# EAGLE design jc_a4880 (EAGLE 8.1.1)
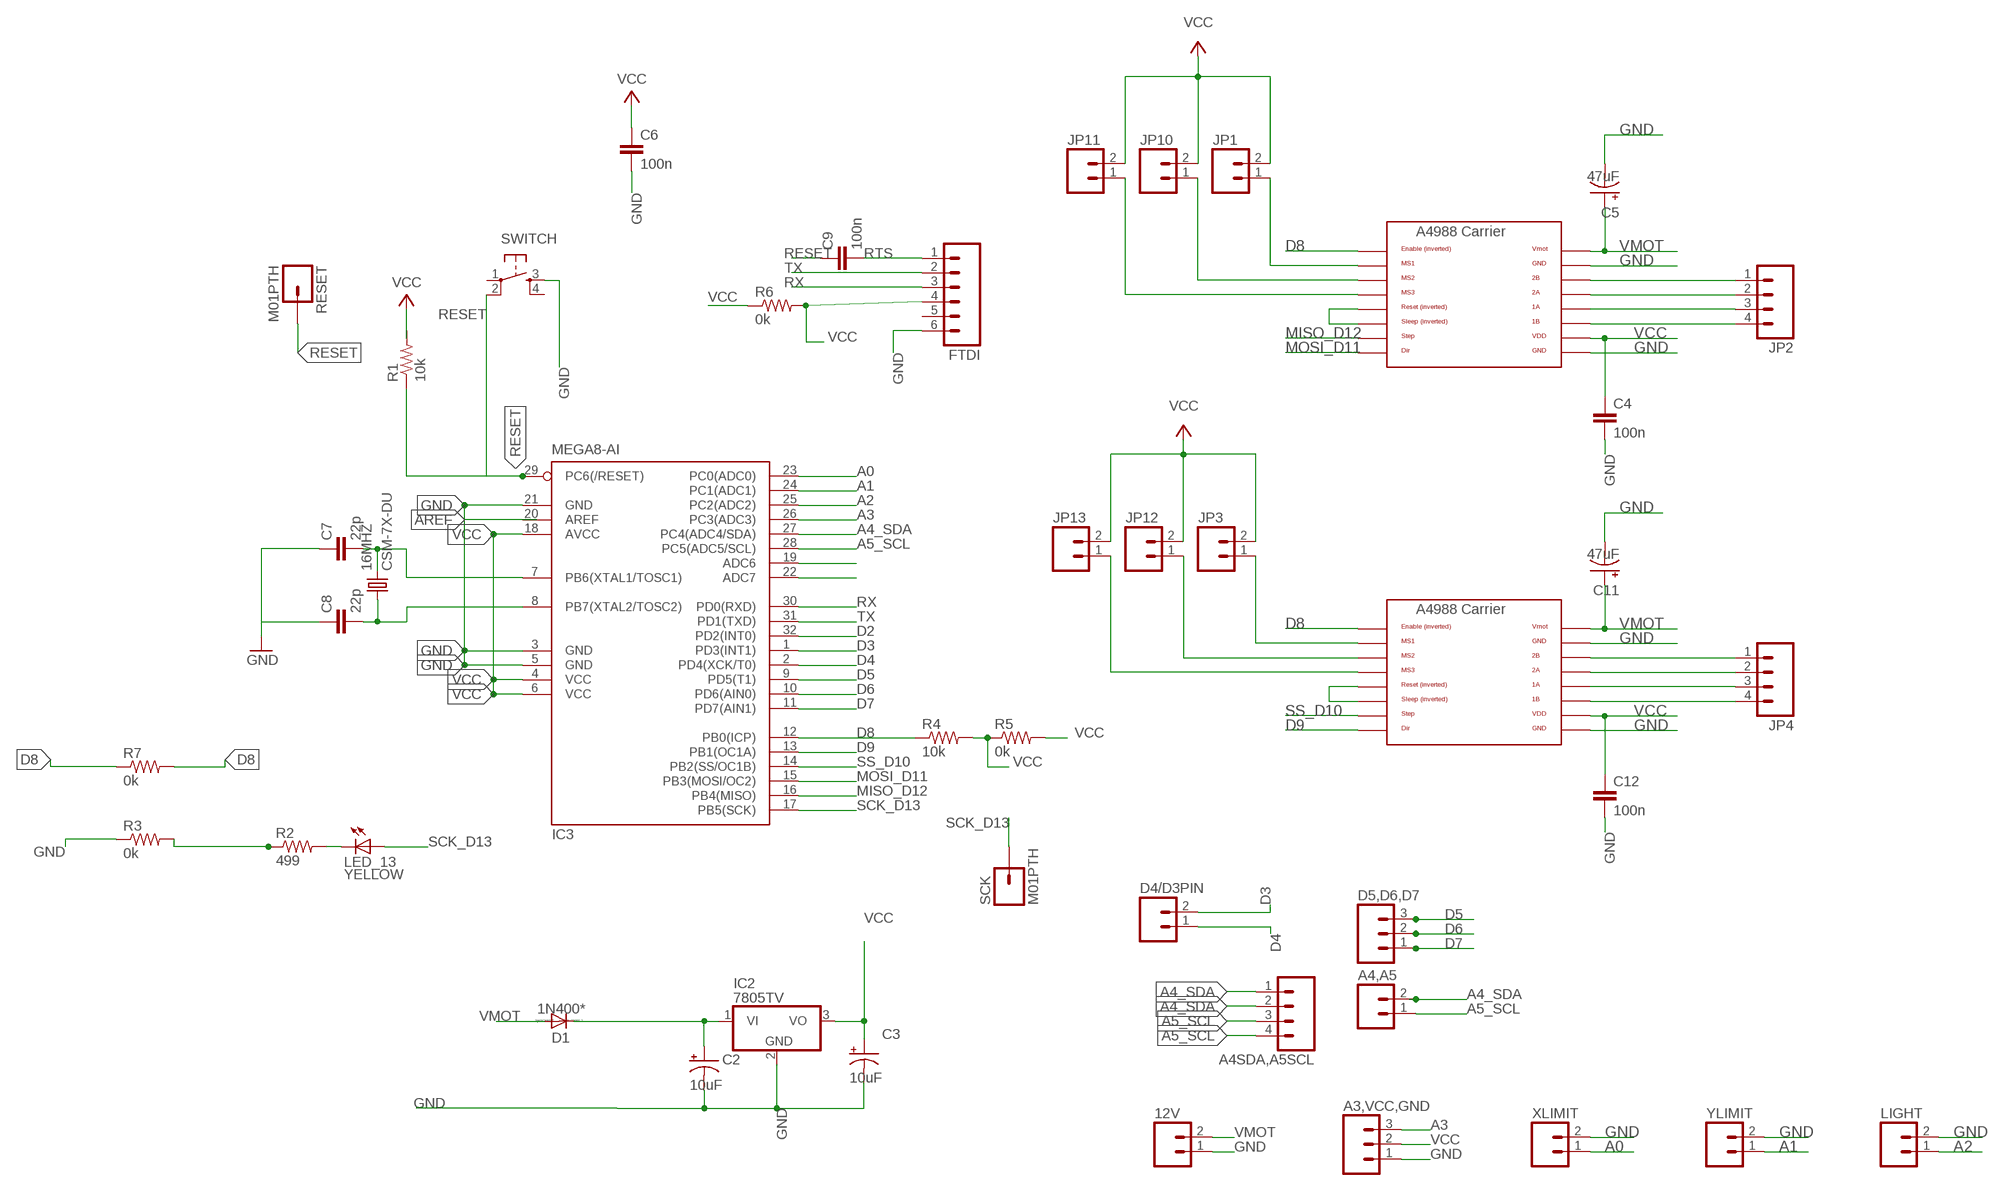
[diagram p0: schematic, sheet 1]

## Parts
12V  M023.5MM_LOCK  [SCREWTERMINAL-3.5MM-2_LOCK]
16MHZ  CSM-7X-DU  [CSM-7X-DU]
A3,VCC,GND  M03PTH  [1X03]
A4,A5  M02PTH  [1X02]
A4SDA,A5SCL  M04PTH  [1X04]
C2  10uF  MCGPR50V107M8X11  [MCGPR50V107M8X11]
C3  10uF  MCGPR50V107M8X11  [MCGPR50V107M8X11]
C4  100n  CAP1206  [1206]
C5  47uF  MCGPR50V107M8X11  [MCGPR50V107M8X11]
C6  100n  CAP1206  [1206]
C7  22p  CAP1206  [1206]
C8  22p  CAP1206  [1206]
C9  100n  CAP1206  [1206]
C11  47uF  MCGPR50V107M8X11  [MCGPR50V107M8X11]
C12  100n  CAP1206  [1206]
D1  1N400*  1N4148DO35-10  [DO35-10]
D4/D3PIN  M02PTH  [1X02]
D5,D6,D7  M03PTH  [1X03]
FTDI  M06LONGPADS  [1X06_LONGPADS]
IC2  7805TV  [TO220V]
IC3  MEGA8-AI  [TQFP32-08]
JP1  M02PTH  [1X02]
JP2  M04PTH  [1X04]
JP3  M02PTH  [1X02]
JP4  M04PTH  [1X04]
JP10  M02PTH  [1X02]
JP11  M02PTH  [1X02]
JP12  M02PTH  [1X02]
JP13  M02PTH  [1X02]
LED_13  YELLOW  LED1206  [1206]
LIGHT  M02LOCK_LONGPADS  [1X02_LOCK_LONGPADS]
R1  10k  RESISTOR1206  [1206]
R2  499  RESISTOR1206  [1206]
R3  0k  RESISTOR1206  [1206]
R4  10k  RESISTOR1206  [1206]
R5  0k  RESISTOR1206  [1206]
R6  0k  RESISTOR1206  [1206]
R7  0k  RESISTOR1206  [1206]
RESET  M01PTH  [1X01]
SCK  M01PTH  [1X01]
SWITCH  6MM_SWITCH6MM_SWITCH  [6MM_SWITCH]
XAXIS  A4988BREAKOUT  [A4988BREAKOUT]
XLIMIT  M02LOCK_LONGPADS  [1X02_LOCK_LONGPADS]
YAXIS1  A4988BREAKOUT  [A4988BREAKOUT]
YLIMIT  M02LOCK_LONGPADS  [1X02_LOCK_LONGPADS]

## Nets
A0: IC3.23(PC0(ADC0)) XLIMIT.1
A1: IC3.24(PC1(ADC1)) YLIMIT.1
A2: IC3.25(PC2(ADC2)) LIGHT.1
A3: A3,VCC,GND.3 IC3.26(PC3(ADC3))
A4_SDA: A4,A5.2 A4SDA,A5SCL.1 A4SDA,A5SCL.2 IC3.27(PC4(ADC4/SDA))
A5_SCL: A4,A5.1 A4SDA,A5SCL.3 A4SDA,A5SCL.4 IC3.28(PC5(ADC5/SCL))
AREF [aref]: IC3.20(AREF)
D2: IC3.32(PD2(INT0))
D3: D4/D3PIN.2 IC3.1(PD3(INT1))
D4: D4/D3PIN.1 IC3.2(PD4(XCK/T0))
D5: D5,D6,D7.3 IC3.9(PD5(T1))
D6: D5,D6,D7.2 IC3.10(PD6(AIN0))
D7: D5,D6,D7.1 IC3.11(PD7(AIN1))
D8: IC3.12(PB0(ICP)) R4.1 R7.1 R7.2 XAXIS.EN YAXIS1.EN
D9: IC3.13(PB1(OC1A)) YAXIS1.DIR
GND: 12V.1 A3,VCC,GND.1 C2.- C3.- C4.2 C5.- C6.2 C7.1 C8.1 C11.- C12.2 FTDI.6 IC2.2(GND) IC3.3(GND) IC3.5(GND) IC3.21(GND) LIGHT.2 R2.1 R3.1 R3.2 SWITCH.3(S) XAXIS.GND XAXIS.GND@0(GND) XLIMIT.2 YAXIS1.GND YAXIS1.GND@0(GND) YLIMIT.2
MISO_D12: IC3.16(PB4(MISO)) XAXIS.STEP
MOSI_D11: IC3.15(PB3(MOSI/OC2)) XAXIS.DIR
N$2: XAXIS.RST XAXIS.SLP(SLEEP)
N$3: JP1.1 XAXIS.MS1
N$4: JP10.1 XAXIS.MS2
N$5: JP11.1 XAXIS.MS3
N$6: 16MHZ.1 C8.2 IC3.8(PB7(XTAL2/TOSC2))
N$8: 16MHZ.2 C7.2 IC3.7(PB6(XTAL1/TOSC1))
N$9: JP2.1 XAXIS.2B
N$10: JP2.2 XAXIS.2A
N$11: JP2.3 XAXIS.1A
N$12: JP2.4 XAXIS.1B
N$13: YAXIS1.RST YAXIS1.SLP(SLEEP)
N$16: JP13.1 YAXIS1.MS3
N$18: JP4.2 YAXIS1.2A
N$19: JP4.1 YAXIS1.2B
N$20: JP4.3 YAXIS1.1A
N$21: JP4.4 YAXIS1.1B
N$27: LED_13.2(C) R2.2
N$38: IC3.22(ADC7)
N$39: IC3.19(ADC6)
N$54: JP3.1 YAXIS1.MS1
N$55: JP12.1 YAXIS1.MS2
RESET: C9.1 IC3.29(PC6(/RESET)) R1.1 RESET.1 SWITCH.2(P1)
RTS: C9.2 FTDI.1
RX: FTDI.3 IC3.30(PD0(RXD))
SCK_D13: IC3.17(PB5(SCK)) LED_13.1(A) SCK.1
SS_D10: IC3.14(PB2(SS/OC1B)) YAXIS1.STEP
TX: FTDI.2 IC3.31(PD1(TXD))
V_IN [gnd]: C2.+ D1.C IC2.1(VI)
VCC: A3,VCC,GND.2 C3.+ C4.1 C6.1 C12.1 FTDI.4 IC2.3(VO) IC3.4(VCC) IC3.6(VCC) IC3.18(AVCC) JP1.2 JP3.2 JP10.2 JP11.2 JP12.2 JP13.2 R1.2 R4.2 R5.1 R5.2 R6.1 R6.2 XAXIS.VDD YAXIS1.VDD
VMOT: 12V.2 C5.+ C11.+ D1.A XAXIS.VMOT YAXIS1.VMOT
Unconnected: FTDI.5 SWITCH.1(P) SWITCH.4(S1)

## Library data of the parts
12V = 01_SparkFun:M02: Header 2
16MHZ = 01_FAB_Hello:CSM-7X-DU: SMD CRYSTAL; OC_FARNELL: unknown; OC_NEWARK: unknown
A3,VCC,GND D5,D6,D7 = 01_SparkFun:M03: Header 3 Standard 3-pin 0.1" header. Use with straight break away headers (SKU : PRT-00116), right angle break away headers (PRT-00553), swiss pins (PRT-00743), machine pins (PRT-00117), and female headers (PRT-00115). Molex polarized connector foot print use with SKU : PRT-08232 with associated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
A4,A5 D4/D3PIN JP1 JP3 JP10-JP13 LIGHT XLIMIT YLIMIT = SparkFun-Connectors:M02: Header 2
A4SDA,A5SCL JP2 JP4 = SparkFun-Connectors:M04: Header 4 Standard 4-pin 0.1" header. Use with straight break away headers (SKU : PRT-00116), right angle break away headers (PRT-00553), swiss pins (PRT-00743), machine pins (PRT-00117), and female headers (PRT-00115). Molex polarized connector foot print use with SKU : PRT-08231 with associated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
C2 C3 C5 C11 = Ryan:MCGPR50V107M8X11
C4 C6-C9 C12 = 01_SparkFun:CAP: Capacitor
D1 = diode:1N4148: DIODE
FTDI = 01_SparkFun:M06: Header 6 Standard 6-pin 0.1" header. Use with straight break away headers (SKU : PRT-00116), right angle break away headers (PRT-00553), swiss pins (PRT-00743), machine pins (PRT-00117), and female headers (PRT-00115). Molex polarized connector foot print use with SKU : PRT-08094 with associated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
IC2 = linear:78*: Positive VOLTAGE REGULATOR Source: http://cache.national.com/ds/LM/LM78L05.pdf http://www.fairchildsemi.com/ds/LM/LM7805.pdf
IC3 = 01_atmel:MEGA8: MICROCONTROLLER 8 Kbytes FLASH, 1 kbytes SRAM, 512 bytes EEPROM, USART, 6-channel 10 bit ADC, 2-channel 8 bit ADC Pin compatible with Atmega48, ATMega88, ATMega168 Source: avr.lbr
LED_13 = 01_FAB_Hello:LED
R1-R7 = 01_SparkFun:RESISTOR: Resistor
RESET SCK = 01_SparkFun:M01: Header 1
SWITCH = 01_FAB_Hello:6MM_SWITCH: OMRON SWITCH
XAXIS YAXIS1 = RepRapjr:A4988BREAKOUT

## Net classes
0 default: width 0.254 mm, drill 0.254 mm, clearance 0.254 mm
1 power: width 0.254 mm, drill 0.254 mm, clearance 0.254 mm
2 gnd: width 0.254 mm, drill 0.254 mm, clearance 0.254 mm
3 usbvcc: width 0.254 mm, drill 0.254 mm, clearance 0.254 mm
4 aref: width 0.254 mm, drill 0.254 mm, clearance 0.254 mm

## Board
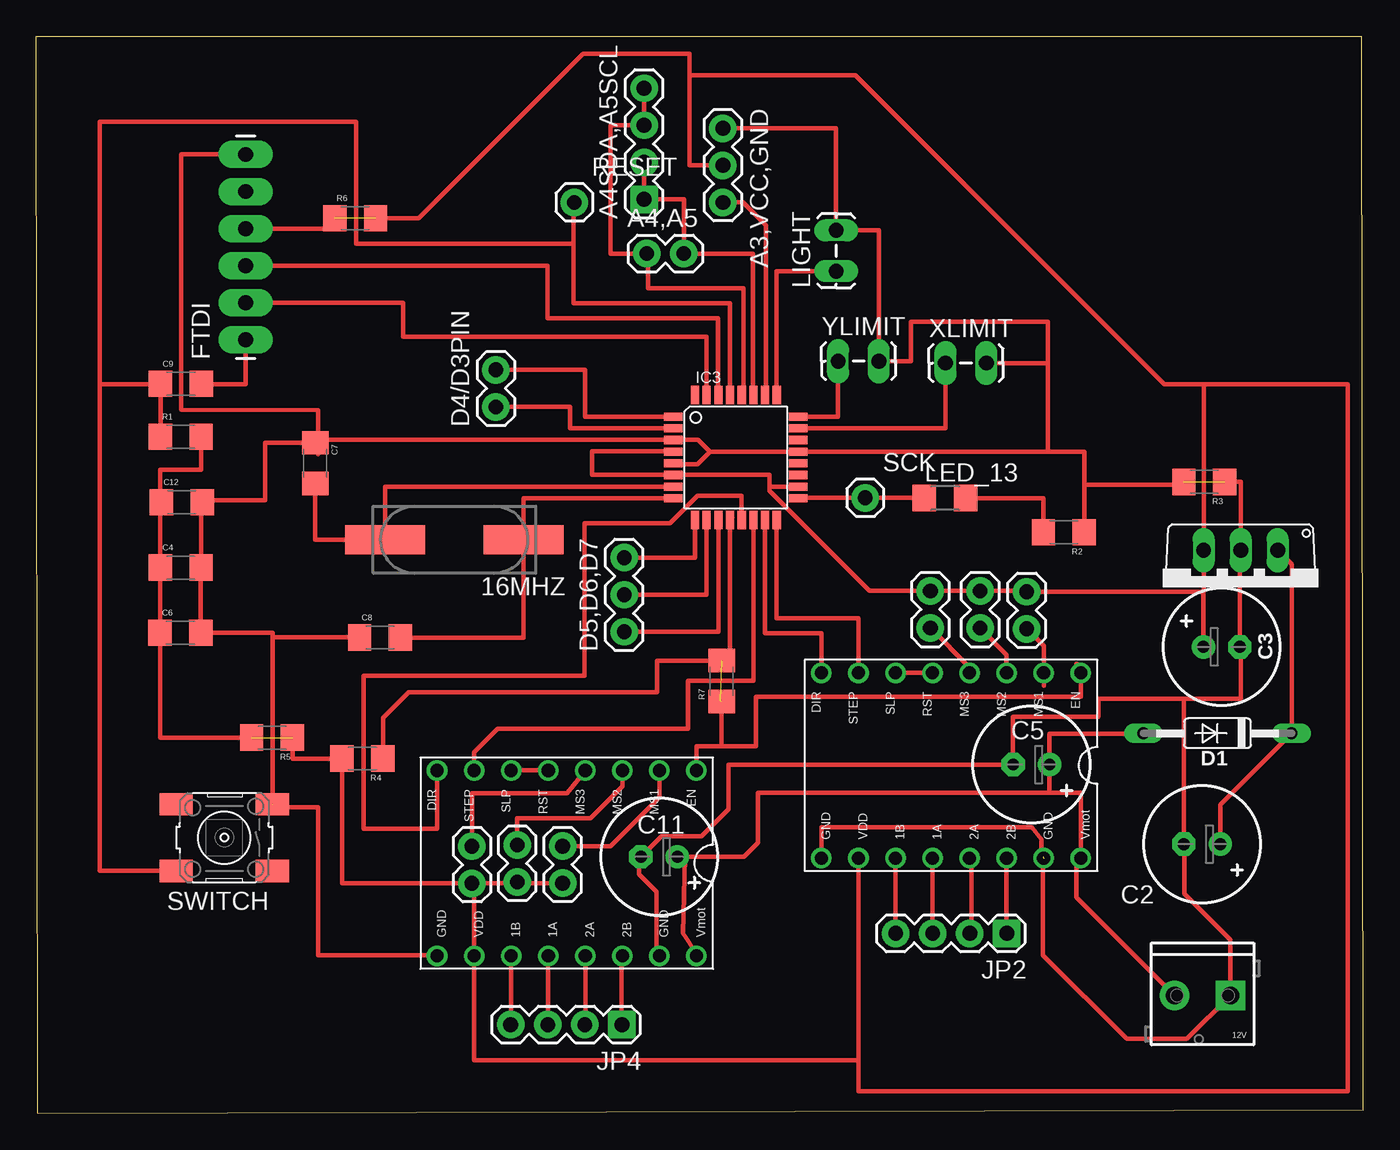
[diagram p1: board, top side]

Size 90.94 x 73.8 mm. Coordinates in mm from the lower left corner, seen from the top.
Outline: 0.09,0 90.94,0.25 90.86,73.8 0,73.8 0.09,0
Copper layers (1*16): Top 0.035mm / dielectric 1.5mm / Bottom 0.035mm
Design rules "default": minimum track width 10mil, minimum drill 24mil, track to track 10mil, track to pad 10mil, pad to pad 10mil, via to via 10mil, smd to smd 10mil, copper to edge 40mil, drill to drill 10mil, minimum pad ring 10mil, minimum via ring 8mil, stop-mask expansion 0mil, vias tented up to drill 0mil, thermal gap 10mil

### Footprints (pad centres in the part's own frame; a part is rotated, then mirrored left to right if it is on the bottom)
SCREWTERMINAL-3.5MM-2_LOCK = drill 1.2 pad 2.032 square: 1 -0.178,0 | drill 1.2 pad 2.032: 2 3.678,0
CSM-7X-DU = smd 5.5 x 2: 1 -4.75,0; 2 4.75,0
1X03 = drill 1.016 pad 1.88: 1 0,0; 2 2.54,0; 3 5.08,0
1X02 = drill 1.016 pad 1.88: 1 0,0; 2 2.54,0
1X04 = drill 1.016 pad 1.88 square: 1 0,0 | drill 1.016 pad 1.88: 2 2.54,0; 3 5.08,0; 4 7.62,0
MCGPR50V107M8X11 = drill 0.813 pad 1.6: + -1.25,0 | drill 0.813 pad 1.6 octagon: - 1.25,0
1206 = smd 1.6 x 1.8: 1 -1.4,0; 2 1.4,0
DO35-10 = drill 0.813 long: A 5.08,0; C -5.08,0
1X06_LONGPADS = drill 1.016 pad 1.88 long: 1 0,0; 2 2.54,0; 3 5.08,0; 4 7.62,0; 5 10.16,0; 6 12.7,0
TO220V = drill 1.016 long: 1 -2.54,-2.54; 2 0,-2.54; 3 2.54,-2.54
TQFP32-08 = smd 1.27 x 0.559: 1 -4.293,2.8; 2 -4.293,2; 3 -4.293,1.2; 4 -4.293,0.4; 5 -4.293,-0.4; 6 -4.293,-1.2; 7 -4.293,-2; 8 -4.293,-2.8; 17 4.293,-2.8; 18 4.293,-2; 19 4.293,-1.2; 20 4.293,-0.4; 21 4.293,0.4; 22 4.293,1.2; 23 4.293,2; 24 4.293,2.8 | smd 0.559 x 1.27: 9 -2.8,-4.293; 10 -2,-4.293; 11 -1.2,-4.293; 12 -0.4,-4.293; 13 0.4,-4.293; 14 1.2,-4.293; 15 2,-4.293; 16 2.8,-4.293; 25 2.8,4.293; 26 2,4.293; 27 1.2,4.293; 28 0.4,4.293; 29 -0.4,4.293; 30 -1.2,4.293; 31 -2,4.293; 32 -2.8,4.293
1206' = smd 1.6 x 1.803: 1 -1.422,0; 2 1.422,0
1X02_LOCK_LONGPADS = drill 1.016 long: 1 -0.127,0; 2 2.667,0
1X01 = drill 1.016 pad 1.88: 1 0,0
6MM_SWITCH = smd 2.286 x 1.524: 1 -3.302,2.286; 2 3.302,2.286; 3 -3.302,-2.286; 4 3.302,-2.286
A4988BREAKOUT = drill 0.9: 1A 8.89,1.27; 1B 11.43,1.27; 2A 6.35,1.27; 2B 3.81,1.27; DIR 16.51,-11.43; EN -1.27,-11.43; GND 16.51,1.27; GND@0 1.27,1.27; MS1 1.27,-11.43; MS2 3.81,-11.43; MS3 6.35,-11.43; RST 8.89,-11.43; SLP 11.43,-11.43; STEP 13.97,-11.43; VDD 13.97,1.27; VMOT -1.27,1.27

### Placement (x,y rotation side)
12V  81.69,8.09 180 top
16MHZ  28.65,39.31 180 top
A3,VCC,GND  47.06,67.5 270 top
A4,A5  41.84,58.92 0 top
A4SDA,A5SCL  41.66,62.63 90 top
C2  79.91,18.45 180 top
C3  81.25,31.97 0 top
C4  9.89,37.41 0 top
C5  68.21,23.9 180 top
C6  9.87,32.94 0 top
C7  19.12,44.56 270 top
C8  23.55,32.61 0 top
C9  9.91,49.99 0 top
C11  42.69,17.58 180 top
C12  9.97,41.89 0 top
D1  80.97,26.04 180 top
D4/D3PIN  31.5,48.41 90 top
D5,D6,D7  40.29,33 90 top
FTDI  14.34,53.01 90 top
IC2  82.55,36.05 180 top
IC3  47.95,44.95 0 top
JP1  67.88,33.2 90 top
JP2  66.52,12.34 180 top
JP3  36.07,18.32 270 top
JP4  40.13,6.08 180 top
JP10  64.7,33.26 90 top
JP11  61.28,33.26 90 top
JP12  32.96,18.39 270 top
JP13  29.85,18.3 270 top
LED_13  YELLOW  [1206']  62.29,42.16 0 top
LIGHT  54.82,57.84 90 top
R1  9.89,46.37 0 top
R2  70.43,39.83 180 top
R3  80.06,43.27 180 top
R4  22.35,24.32 180 top
R5  16.15,25.75 180 top
R6  21.85,61.35 0 top
R7  46.98,29.62 90 top
RESET  36.88,62.43 0 top
SCK  56.82,42.18 0 top
SWITCH  12.88,18.9 180 top
XAXIS  70.32,18.76 180 top
XLIMIT  62.45,51.42 0 top
YAXIS1  43.98,12.07 180 top
YLIMIT  55.09,51.55 0 top

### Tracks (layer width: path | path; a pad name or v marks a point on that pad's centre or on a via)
A0
  Top 0.305: 52.29,47 IC3.23 62.32,46.95 XLIMIT.1
A1
  Top 0.305: IC3.24 54.96,47.75 YLIMIT.1
A2
  Top 0.305: 50.91,48.8 IC3.25 50.75,57.72 LIGHT.1
A3
  Top 0.305: IC3.26 50.01,49.31 50.01,60.85 48.43,62.42 A3,VCC,GND.3
A4_SDA
  Top 0.305: IC3.27 49.11,49.28 49.11,58.92 A4,A5.2 44.38,62.63 A4SDA,A5SCL.1 A4SDA,A5SCL.2
A5_SCL
  Top 0.254: IC3.28 48.41,49.31
  Top 0.305: IC3.28 48.46,49.36 48.46,56.54 41.91,56.54 41.91,58.92 A4,A5.1 39.37,58.92 39.37,67.71 A4SDA,A5SCL.3 A4SDA,A5SCL.4
D3
  Top 0.305: IC3.1 37.59,47.75 37.59,50.95 D4/D3PIN.2
D4
  Top 0.305: IC3.2 36.58,46.95 36.58,48.41 D4/D3PIN.1
D5
  Top 0.305: IC3.9 45.15,38.08 D5,D6,D7.3
D6
  Top 0.305: IC3.10 45.95,35.54 D5,D6,D7.2
D7
  Top 0.305: IC3.11 46.75,33 D5,D6,D7.1
D8  (2 unrouted)
  Top 0.305: 71.31,30.8 XAXIS.EN 71.59,28.55 49.33,28.55 49.33,25.15 46.98,25.15 | 47.71,40.82 IC3.12 47.55,31.02 R7.2 42.55,31.02 42.55,28.86 25.51,28.86 23.75,27.1 R4.1 | YAXIS1.EN 45.25,25.15 46.98,25.15 | 46.86,28.28 46.89,28.28 | R7.1 46.98,25.15
D9
  Top 0.305: 48.36,40.65 IC3.13 48.35,42.33 45.32,42.33 43.43,40.43 37.57,40.43 37.57,30 22.42,30 22.42,19.52 27.47,19.52 YAXIS1.DIR 27.47,23.86
GND  (5 unrouted)
  Top 0.305: C7.1 19.3,45.16 19.3,48.18 9.92,48.22 9.92,65.71 FTDI.6 | 46.16,45.35 IC3.21 | 46.16,45.35 45.31,44.5 43.71,44.5 IC3.5 | 46.16,45.35 45.36,46.15 IC3.3 19.12,46.15 C7.1 | 52.29,45.3 IC3.21 | XLIMIT.2 69.34,51.42 | 69.34,45.35 IC3.21 | 69.34,51.42 69.34,45.35 | A3,VCC,GND.1 54.82,67.5 LIGHT.2 57.75,60.51 YLIMIT.2 59.94,51.55 59.94,54.25 69.34,54.25 69.34,51.42 | 69.34,45.35 71.83,45.35 71.83,43.08 | C8.1 16.2,32.61 | 16.2,32.61 16.2,21.18 | 78.66,28.4 82.55,28.4 82.55,31.97 C3.- 82.5,38.59 IC2.2 82.55,43.27 R3.1 | C2.- 78.66,28.4 | 71.83,43.08 R2.1 | C11.- 42.85,19 45.61,19 47.46,20.85 47.46,23.9 C5.- 66.96,27.17 72.79,27.17 72.79,28.4 78.66,28.4 | 42.51,10.6 42.51,15.2 41.31,16.4 41.31,17.6 | 42.86,10.45 42.51,10.4 42.51,10.6 | 42.51,10.6 42.58,10.67 42.71,10.67 YAXIS1.GND@0 | 78.71,18.4 78.71,15.05 81.86,11.9 12V.1 78.88,5.1 74.76,5.1 69.01,10.85 69.01,17.6 68.91,17.6 68.91,18.8 68.26,19.6 53.81,19.6 XAXIS.GND | SWITCH.3 16.18,20.99 19.3,20.99 19.3,10.82 27.47,10.82 YAXIS1.GND | R3.2 78.66,43.08 71.83,43.08 | 16.2,32.61 16.2,32.94 C6.2 11.27,37.41 C4.2 11.29,41.89 C12.2 11.37,42.01 15.69,42.01 15.69,45.96 C7.1
MISO_D12
  Top 0.305: XAXIS.STEP 56.35,33.93 50.75,33.93 IC3.16
MOSI_D11
  Top 0.305: 49.96,40.65 IC3.15 49.95,32.92 53.81,32.92 XAXIS.DIR
N$2
  Top 0.305: XAXIS.SLP XAXIS.RST
N$3
  Top 0.305: 69.06,29.3 XAXIS.MS1 69.05,32.04 JP1.1
N$4
  Top 0.305: XAXIS.MS2 66.51,31.44 JP10.1
N$5
  Top 0.305: XAXIS.MS3 63.97,30.57 JP11.1
N$6
  Top 0.305: C8.2 24.95,32.35 | 24.35,32.61 C8.2 | IC3.8 33.4,42.15 16MHZ.1 33.4,32.61 C8.2
N$8
  Top 0.305: IC3.7 23.89,42.95 16MHZ.2 19.12,39.31 C7.2
N$9
  Top 0.012: 66.51,17.6 XAXIS.2B
  Top 0.305: 66.51,17.6 66.51,12.8 JP2.1
N$10
  Top 0.305: 64.11,17.6 64.11,17.55 | 64.11,17.55 64.11,12.46 JP2.2 | XAXIS.2A 64.05,17.49 64.11,17.55
N$11
  Top 0.305: XAXIS.1A 61.43,12.35 JP2.3
N$12
  Top 0.305: XAXIS.1B 58.89,12.35 JP2.4
N$13
  Top 0.305: YAXIS1.SLP YAXIS1.RST
N$16
  Top 0.305: YAXIS1.MS3 37.71,23.6 36.36,21.95 29.85,21.95 JP13.1
N$18
  Top 0.305: YAXIS1.2A 37.63,6.11 JP4.2
N$19
  Top 0.305: JP4.1 40.11,6.11 40.11,10.74 YAXIS1.2B
N$20
  Top 0.305: YAXIS1.1A 35.09,6.11 JP4.3
N$21
  Top 0.305: YAXIS1.1B 32.55,6.11 JP4.4
N$27
  Top 0.305: 69.03,40.74 R2.2 69.03,42.16 LED_13.2
N$54
  Top 0.305: 36.19,18.44 JP3.1 39.35,18.32 39.36,18.31 42.71,21.66 YAXIS1.MS1
N$55
  Top 0.305: 32.91,18.8 JP12.1 32.96,20.24 38,20.24 40.17,22.4 YAXIS1.MS2 40.11,23.6
RESET
  Top 0.305: 36.83,59.1 36.83,55.52 47.55,55.52 IC3.29 | 36.83,59.1 36.83,59.6 21.9,59.6 21.9,67.96 4.35,67.96 4.35,49.97 | 9.58,16.59 SWITCH.2 4.35,16.61 4.35,49.97 | R1.1 8.51,46.37 C9.1 8.51,49.97 4.35,49.97 | RESET.1 36.83,62.43 36.83,59.1
RTS
  Top 0.305: FTDI.1 14.34,49.96 11.31,49.96 C9.2
RX
  Top 0.305: IC3.30 46.71,49.28 46.71,54.51 35.05,54.51 35.05,58.09 FTDI.3
SCK_D13
  Top 0.305: IC3.17 52.24,42.18 SCK.1 LED_13.1
SS_D10
  Top 0.305: 49.16,40.65 IC3.14 49.15,30.68 | YAXIS1.STEP 30.01,24.75 31.61,26.35 44.66,26.35 44.66,29.64 49.15,29.64 49.15,30.68 | 49.15,30.68 49.15,29.87
TX
  Top 0.305: 45.91,49.28 IC3.31 45.95,53.24 25.15,53.24 25.15,55.55 FTDI.2 14.34,55.52
V_IN
  Top 0.305: IC2.1 86.05,37.64 D1.C 81.16,21.16 C2.+
VCC  (via drill 0.6)  (2 unrouted)
  Top 0.012: IC3.6
  Top 0.305: IC3.4 43.65,45.36 38.1,45.36 38.1,43.75 IC3.6 50.24,43.75 50.24,42.95 | 14.1,26.41 R5.2 8.47,25.75 C6.1 8.47,37.41 C4.1 8.49,41.89 C12.1 8.47,41.89 8.47,44.11 11.29,44.11 R1.2 | 20.45,61.87 R6.1 20.45,60.63 FTDI.4 | 30.01,15.78 YAXIS1.VDD 30.01,3.64 56.35,3.64 | 30.01,15.78 JP3.2 36.07,15.76 20.95,15.76 R4.2 17.55,24.32 R5.1 | JP12.2 32.87,15.76 JP13.2 29.99,15.76 30.01,15.78 | 67.8,35.83 JP1.2 | JP1.2 67.83,35.8 JP10.2 JP11.2 57.09,35.8 50.24,42.66 50.24,42.95 | 80,35.74 JP1.2 | 50.24,42.95 IC3.18 | A3,VCC,GND.2 44.78,64.96 44.78,71.15 | 44.78,71.15 56.14,71.15 77.33,49.95 80.02,49.95 | 56.35,3.64 XAXIS.VDD | 56.35,3.64 56.35,1.52 89.91,1.52 89.91,49.95 80.02,49.95 | C3.+ 80,35.74 | 80,35.74 80.02,35.74 IC2.3 80.02,49.95 | 44.78,71.15 44.78,72.63 37.48,72.63 26.2,61.35 R6.2
  other vias: 80.01,38.59
VMOT
  Top 0.305: YAXIS1.VMOT 45.26,10.95 44.31,12.35 44.46,17.5 C11.+ 43.95,17.6 48.51,17.6 49.46,18.55 49.46,21.97 69.46,21.97 | 68.91,23.6 C5.+ | D1.A 75.84,26 69.46,26 C5.+ | 12V.2 71.31,14.79 71.31,17.6 XAXIS.VMOT 71.59,21.97 69.46,21.97 | 69.46,21.97 C5.+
